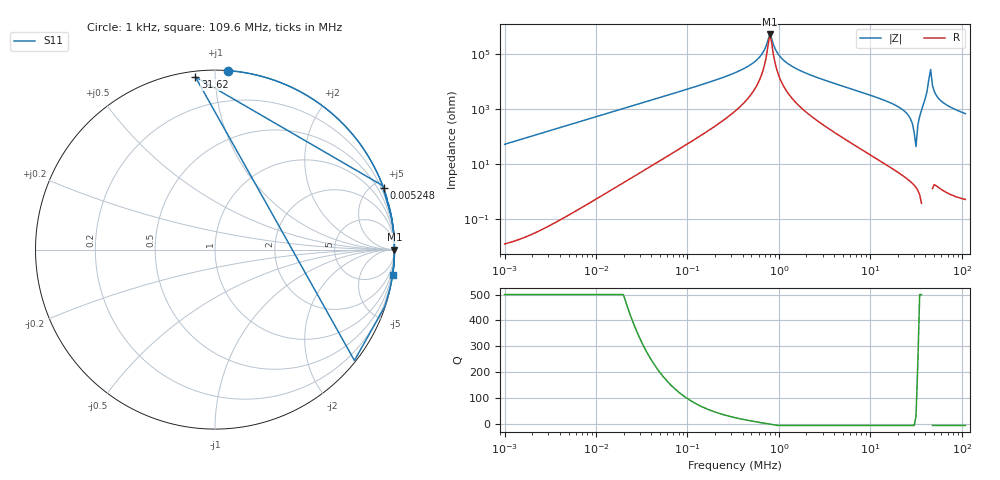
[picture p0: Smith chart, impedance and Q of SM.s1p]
! EM Consulting and Software
! Touchstone file was created on 2026-03-09  16:25:52
# HZ S RI R 50.0000
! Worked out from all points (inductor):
!   253 points, 1 kHz to 109.6 MHz, reference 50 ohm
!   read as one part to ground: L = 8.58 mH near 1.047 kHz
!   highest |Z| = 530 kohm at 794.3 kHz (marker M1)
!   self-resonance near 794.3 kHz
!   S11 on the Smith chart (normalised r, x): 1 kHz: 0.00, +1.08; 5.248 kHz: 0.00, +5.66; 31.62 MHz: 0.03, +0.89; 109.6 MHz: 0, -14
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1000  0.0746 0.997
1202.264  0.2533 0.9672
1445.44  0.4162 0.909
1995.262  0.6442 0.7646
2884.032  0.8122 0.583
4365.158  0.9134 0.4067
5248.075  0.9392 0.3428
9120.108  0.9793 0.2014
18197.01  0.9946 0.1017
34673.69  0.9984 0.0534
79432.82  0.9995 0.0231
331131.1  0.9998 0.00464
794328.2  0.9998 3.34e-05
1445440  0.9998 -0.00291
6025596  0.9997 -0.0175
1.819701e7  0.9975 -0.0665
2.290868e7  0.994 -0.1057
2.630268e7  0.9847 -0.1697
2.754229e7  0.9746 -0.2187
2.884032e7  0.9459 -0.3178
3.019952e7  0.7767 -0.6178
3.162278e7  -0.1094 0.9621
3.311311e7  0.9323 0.3576
3.467369e7  0.9836 0.179
3.630781e7  0.9943 0.1065
3.801894e7  0.9978 0.0667
4.365158e7  1 0.00814
1.096478e8  0.9897 -0.1423
